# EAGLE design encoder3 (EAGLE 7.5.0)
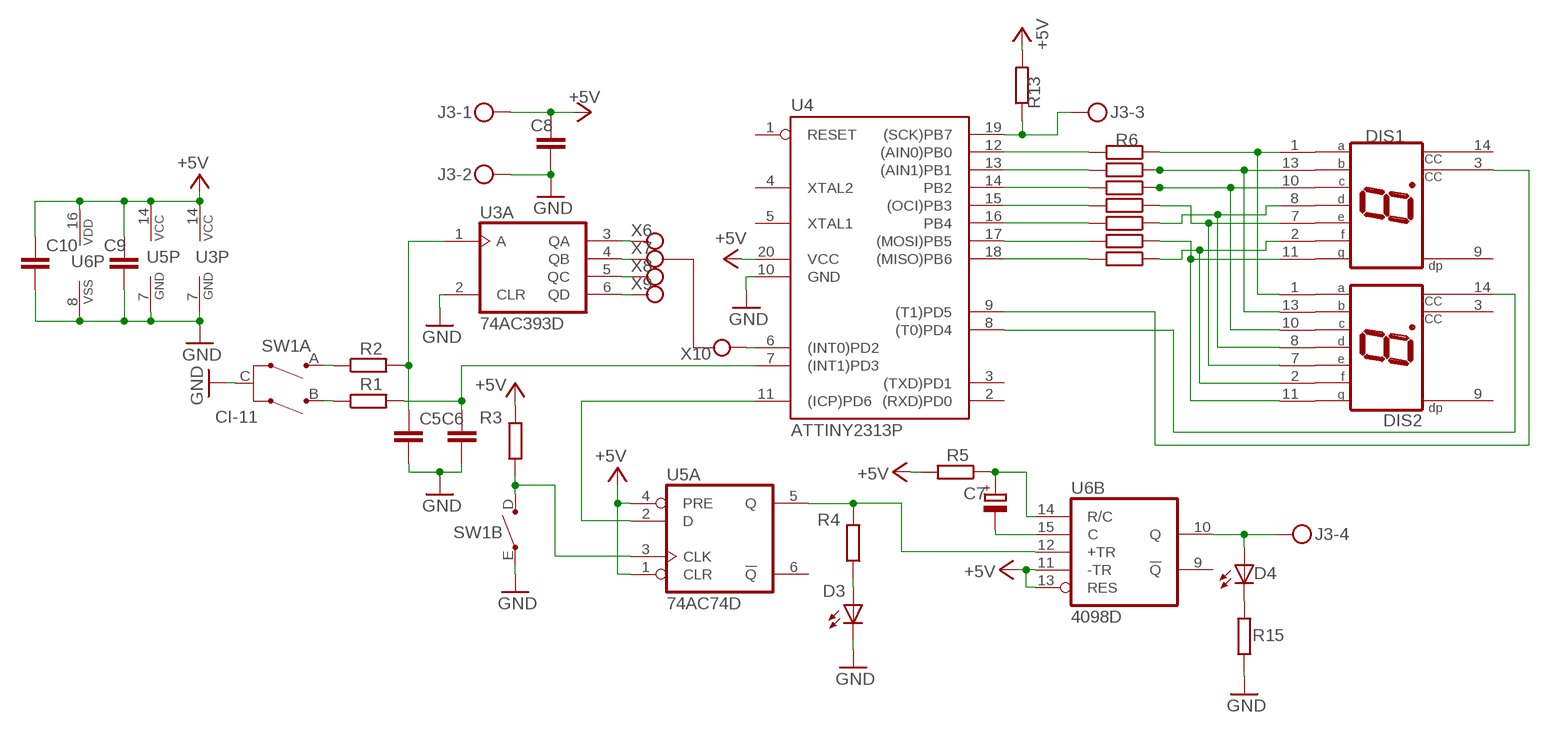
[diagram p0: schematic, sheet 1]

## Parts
C5  C-EUC1206  [C1206]
C6  C-EUC1206  [C1206]
C7  CPOL-EUE2.5-5  [E2,5-5]
C8  C-EUC1206  [C1206]
C9  C-EUC1206  [C1206]
C10  C-EUC1206  [C1206]
D3  LED3MM  [LED3MM]
D4  LED3MM  [LED3MM]
DIS1  VAOS-C402S9-BW/50  HD7740  [HD7730]
DIS2  VAOS-C402S9-BW/50  HD7740  [HD7730]
J3  MKDSN1,5/4-5,08  [MKDSN1,5/4-5,08]
R1  R-EU_0204/7  [0204/7]
R2  R-EU_0204/7  [0204/7]
R3  R-EU_0204/7  [0204/7]
R4  R-EU_0204/7  [0204/7]
R5  R-EU_0204/5  [0204/5]
R6  R-EU_0204/7  [0204/7]
R7  R-EU_0204/7  [0204/7]
R8  R-EU_0204/7  [0204/7]
R9  R-EU_0204/7  [0204/7]
R10  R-EU_0204/7  [0204/7]
R11  R-EU_0204/7  [0204/7]
R12  R-EU_0204/7  [0204/7]
R13  R-EU_0204/7  [0204/7]
R15  R-EU_0204/7  [0204/7]
SW1  CI-11  [CI-11]
U3  74AC393D  [SO14]
U4  ATTINY2313P  AT90S2313P  [DIL20]
U5  74AC74D  [SO14]
U6  4098D  [SO16]
X6  CONNWIRE  [CONNWIRE]
X7  CONNWIRE  [CONNWIRE]
X8  CONNWIRE  [CONNWIRE]
X9  CONNWIRE  [CONNWIRE]
X10  CONNWIRE  [CONNWIRE]

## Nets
+5V: C8.1 C9.1 C10.1 J3.1 R3.2 R5.2 R13.2 U3.14(P:VCC) U4.20(VCC) U5.1(A:CLR) U5.4(A:PRE) U5.14(P:VCC) U6.11(B:-TR) U6.13(B:RES) U6.16(P:VDD)
GND: C5.2 C6.2 C8.2 C9.2 C10.2 D3.K(C) J3.2 R15.1 SW1.C(A:C) SW1.E(B:E) U3.2(A:CLR) U3.7(P:GND) U4.10(GND) U5.7(P:GND) U6.8(P:VSS)
N$2: J3.3 R13.1 U4.19((SCK)PB7)
N$3: R2.1 SW1.A(A:A)
N$4: D4.A J3.4 U6.10(B:Q)
N$5: R1.1 SW1.B(A:B)
N$6: R6.2 U4.12((AIN0)PB0)
N$7: D4.K(C) R15.2
N$8: R7.2 U4.13((AIN1)PB1)
N$9: R8.2 U4.14(PB2)
N$10: R9.2 U4.15((OCI)PB3)
N$11: R10.2 U4.16(PB4)
N$12: DIS1.1(A) DIS2.1(A) R6.1
N$13: C6.1 R1.2 U4.7((INT1)PD3)
N$14: C5.1 R2.2 U3.1(A:A)
N$15: U3.3(A:QA) X6.P$1
N$16: U3.4(A:QB) X7.P$1
N$17: U3.5(A:QC) X8.P$1
N$18: U3.6(A:QD) X9.P$1
N$19: U4.6((INT0)PD2) X10.P$1
N$20: U4.11((ICP)PD6) U5.2(A:D)
N$21: R3.1 SW1.D(B:D) U5.3(A:CLK)
N$22: R12.2 U4.18((MISO)PB6)
N$23: DIS1.13(B) DIS2.13(B) R7.1
N$24: R4.2 U5.5(A:Q) U6.12(B:+TR)
N$25: D3.A R4.1
N$26: C7.+ R5.1 U6.14(B:R/C)
N$27: C7.- U6.15(B:C)
N$28: DIS1.10(C) DIS2.10(C) R8.1
N$29: DIS1.7(E) DIS2.7(E) R9.1
N$30: DIS1.8(D) DIS2.8(D) R10.1
N$32: DIS1.11(G) DIS2.11(G) R11.1
N$33: DIS1.2(F) DIS2.2(F) R12.1
N$34: R11.2 U4.17((MOSI)PB5)
N$35: DIS2.14(CC) U4.8((T0)PD4)
N$51: DIS1.3(CC) U4.9((T1)PD5)
Unconnected: DIS1.9(DP) DIS1.14(CC) DIS2.3(CC) DIS2.9(DP) U3.8(B:QD) U3.9(B:QC) U3.10(B:QB) U3.11(B:QA) U3.12(B:CLR) U3.13(B:A) U4.1(RESET) U4.2((RXD)PD0) U4.3((TXD)PD1) U4.4(XTAL2) U4.5(XTAL1) U5.6(A:!Q) U5.8(B:!Q) U5.9(B:Q) U5.10(B:PRE) U5.11(B:CLK) U5.12(B:D) U5.13(B:CLR) U6.1(A:C) U6.2(A:R/C) U6.3(A:RES) U6.4(A:+TR) U6.5(A:-TR) U6.6(A:Q) U6.7(A:!Q) U6.9(B:!Q)

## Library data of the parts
C5 C6 C8-C10 = rcl:C-EU: CAPACITOR, European symbol
C7 = rcl:CPOL-EU: POLARIZED CAPACITOR, European symbol
D3 D4 = led:LED: LED
DIS1 DIS2 = display-hp:HD7740: LED DISPLAY 1-character 7 segment, decimal point right; OC_FARNELL: unknown; OC_NEWARK: unknown
J3 = con-phoenix-508:MKDSN1,5/4-5,08: MKDSN 1,5/ 4-5,08 Printklemme Nennstrom: 13,5 A Nennspannung: 250 V Rastermaß: 5,08 mm Polzahl: 4 Anschlussart: Schraubanschluss Montage: Löten Anschlussrichtung Leiter/Platine: 0 ° Artikelnummer: 1729144 Source: http://eshop.phoenixcontact.com .. 1729144.pdf
R1-R13 R15 = rcl:R-EU_: RESISTOR, European symbol
SW1 = piher:CI-11: 11mm Incemental Encoder Source: www.piher.net .. 04-CI-11v04.pdf; OC_FARNELL: unknown; OC_NEWARK: unknown
U3 = 74xx-eu:74*393: Dual 4-bit decade and binary COUNTER
U4 = atmel:AT90S2313: MICROCONTROLLER 2 Kbytes FLASH 128 bytes SRAM 128 bytes EEPROM UART; OC_FARNELL: unknown; OC_NEWARK: unknown
U5 = 74xx-eu:74*74: Dual D type positive edge triggered FLIP FLOP, preset and clear
U6 = 40xx:4098: Dual monostable MULTIVIBRATOR Source: Texas Instruments (Data sheet acquired frm Harris Semiconductor SCHS065) http://pdf1.alldatasheet.com/datasheet-pdf/view/26897/TI/CD4098.html
X6-X10 = connholes:CONNWIRE

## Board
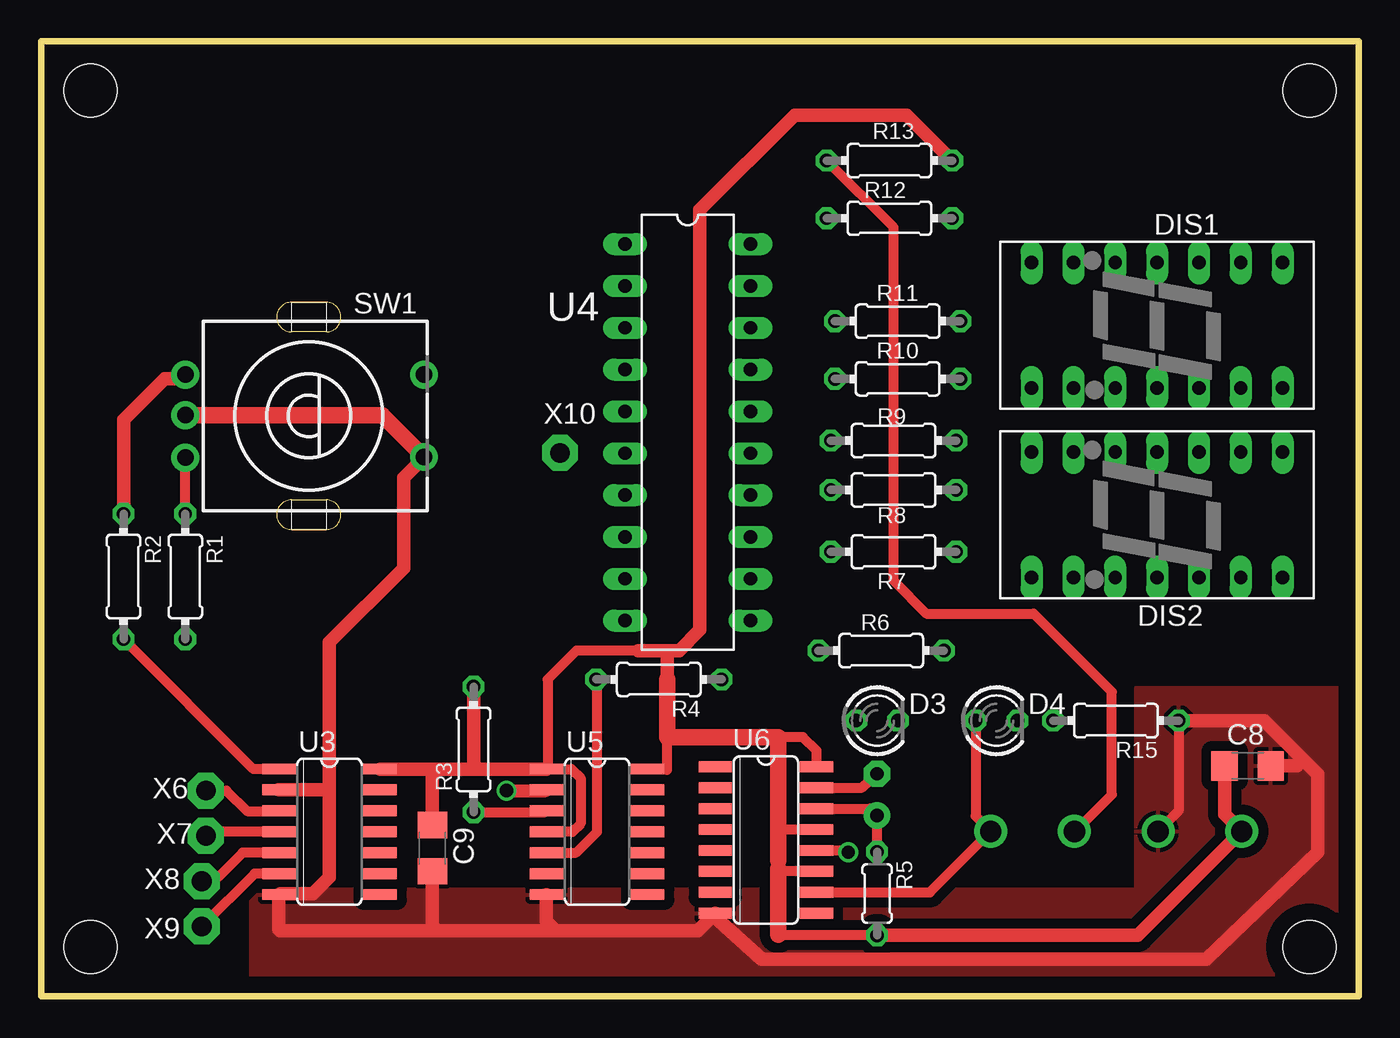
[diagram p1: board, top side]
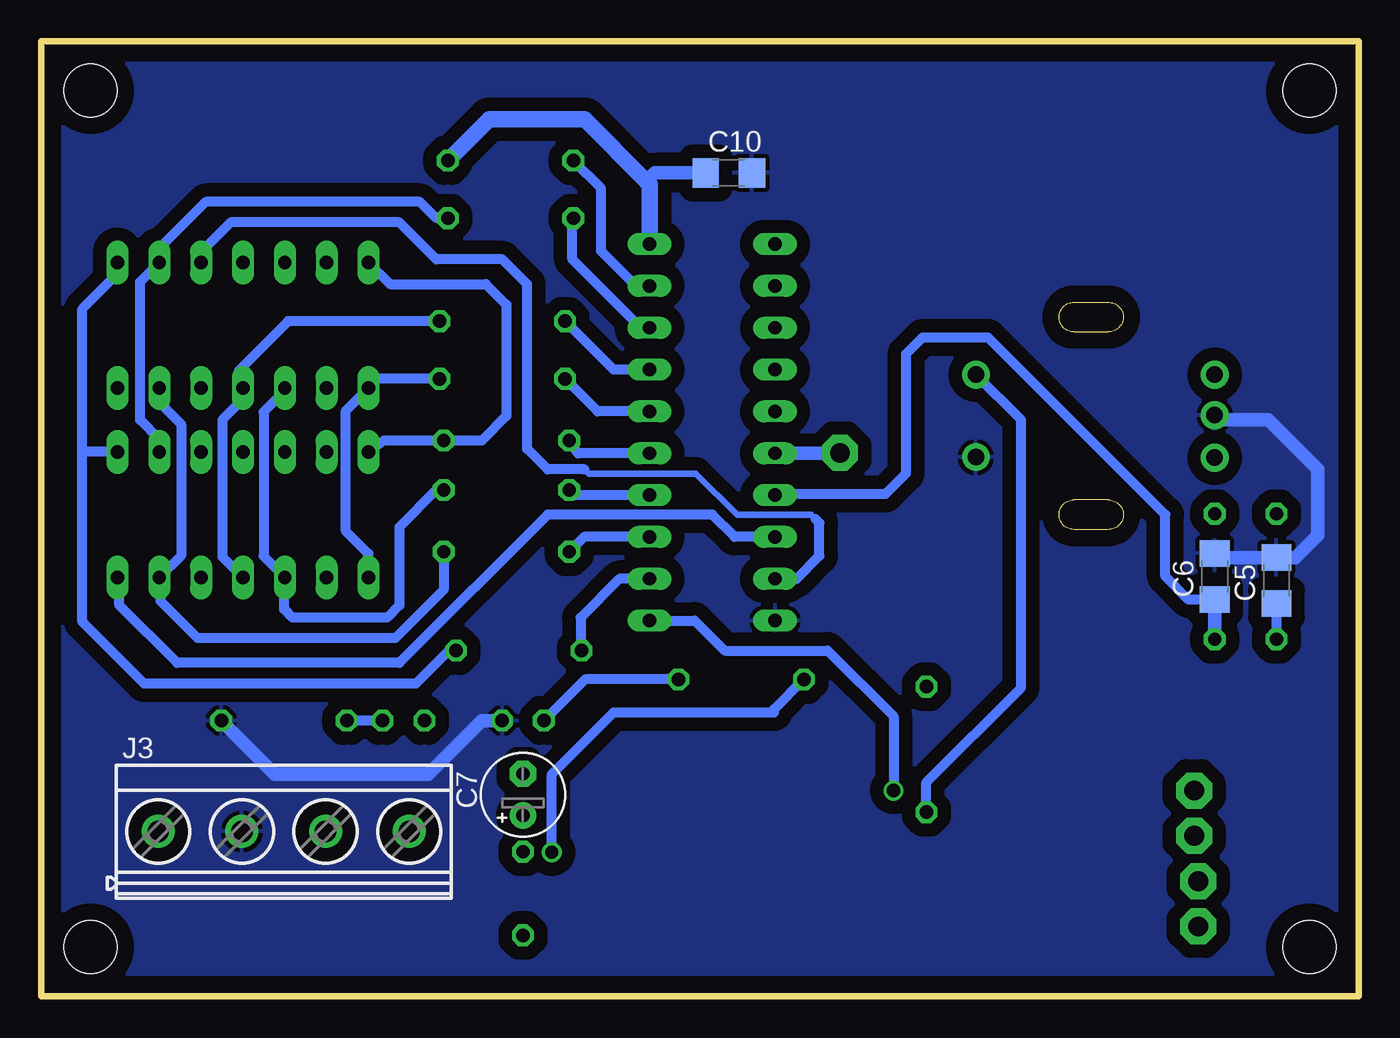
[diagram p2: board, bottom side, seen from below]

Size 80 x 58 mm. Coordinates in mm from the lower left corner, seen from the top.
Outline: 0,0 0,58 80,58 80,0 0,0
Copper layers (1*16): Top 0.035mm / dielectric 1.5mm / Bottom 0.035mm
Design rules "default": minimum track width 10mil, minimum drill 24mil, track to track 8mil, track to pad 8mil, pad to pad 8mil, via to via 8mil, smd to smd 8mil, copper to edge 40mil, drill to drill 8mil, minimum pad ring 10mil, minimum via ring 8mil, stop-mask expansion 4mil, vias tented up to drill 0mil, thermal gap 10mil
Holes 3.2 mm at 3,3 3,55 77,55 77,3

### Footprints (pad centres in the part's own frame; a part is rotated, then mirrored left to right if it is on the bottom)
C1206 = smd 1.6 x 1.8: 1 -1.4,0; 2 1.4,0
E2,5-5 = drill 0.813 pad 1.6: + -1.27,0 | drill 0.813 pad 1.6 octagon: - 1.27,0
LED3MM = drill 0.813 octagon: A -1.27,0; K 1.27,0
HD7730 = drill 0.813 long: 1 -3.81,7.62; 2 -3.81,5.08; 3 -3.81,2.54; 4 -3.81,0; 5 -3.81,-2.54; 6 -3.81,-5.08; 7 -3.81,-7.62; 8 3.81,-7.62; 9 3.81,-5.08; 10 3.81,-2.54; 11 3.81,0; 12 3.81,2.54; 13 3.81,5.08; 14 3.81,7.62
MKDSN1,5/4-5,08 = drill 1.3 pad 2: 1 -7.641,0.025; 2 -2.561,0.025; 3 2.519,0.025; 4 7.599,0.025
0204/7 = drill 0.813 octagon: 1 -3.81,0; 2 3.81,0
0204/5 = drill 0.813 octagon: 1 -2.54,0; 2 2.54,0
CI-11 = drill 1 pad 1.676: A -2.5,-7.5; B 2.54,-7.5; C -0.04,-7.5; D -2.5,7; E 2.5,7
SO14 = smd 0.66 x 2.032: 1 -3.81,-3.073; 2 -2.54,-3.073; 3 -1.27,-3.073; 4 0,-3.073; 5 1.27,-3.073; 6 2.54,-3.073; 7 3.81,-3.073; 8 3.81,3.073; 9 2.54,3.073; 10 1.27,3.073; 11 0,3.073; 12 -1.27,3.073; 13 -2.54,3.073; 14 -3.81,3.073
DIL20 = drill 0.813 long: 1 -11.43,-3.81; 2 -8.89,-3.81; 3 -6.35,-3.81; 4 -3.81,-3.81; 5 -1.27,-3.81; 6 1.27,-3.81; 7 3.81,-3.81; 8 6.35,-3.81; 9 8.89,-3.81; 10 11.43,-3.81; 11 11.43,3.81; 12 8.89,3.81; 13 6.35,3.81; 14 3.81,3.81; 15 1.27,3.81; 16 -1.27,3.81; 17 -3.81,3.81; 18 -6.35,3.81; 19 -8.89,3.81; 20 -11.43,3.81
SO16 = smd 0.66 x 2.032: 1 -4.445,-3.073; 2 -3.175,-3.073; 3 -1.905,-3.073; 4 -0.635,-3.073; 5 0.635,-3.073; 6 1.905,-3.073; 7 3.175,-3.073; 8 4.445,-3.073; 9 4.445,3.073; 10 3.175,3.073; 11 1.905,3.073; 12 0.635,3.073; 13 -0.635,3.073; 14 -1.905,3.073; 15 -3.175,3.073; 16 -4.445,3.073
CONNWIRE = drill 1.2 pad 2.184 octagon: P$1 0,0

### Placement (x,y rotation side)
C5  5,25.25 90 bottom
C6  8.75,25.5 90 bottom
C7  50.75,12.25 90 bottom
C8  73.25,14 0 top
C9  23.75,9 270 top
C10  38.25,50 0 bottom
D3  50.75,16.75 0 top
D4  58,16.75 0 top
DIS1  67.75,40.75 270 top
DIS2  67.75,29.25 270 top
J3  65.25,10 0 bottom
R1  8.75,25.5 270 top
R2  5,25.5 270 top
R3  26.25,15 90 top
R4  37.5,19.25 180 top
R5  50.75,6.25 270 top
R6  51,21 180 top
R7  51.75,27 180 top
R8  51.75,30.75 180 top
R9  51.75,33.75 180 top
R10  52,37.5 180 top
R11  52,41 180 top
R12  51.5,47.25 180 top
R13  51.5,50.75 0 top
R15  65.25,16.75 180 top
SW1  16.25,35.25 270 top
U3  17.5,10 270 top
U4  39.25,34.25 270 top
U5  33.75,10 270 top
U6  44,9.5 270 top
X6  10,12.5 0 top
X7  10,9.75 0 top
X8  9.75,7 0 top
X9  9.75,4.25 0 top
X10  31.5,33 0 top

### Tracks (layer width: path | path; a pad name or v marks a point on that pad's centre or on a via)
+5V
  Top 0.61: U6.16 47.07,14.93 46.25,15.75 44.75,15.75 | 38,15.75 38.25,15.75 38,15.5 38,13.75 37.94,13.81 U5.14 | 36.25,21 32.5,21 30.75,19.25 30.75,13.88 U5.1 32.19,13.81 32.75,13.25 32.75,10.5 32.25,10 U5.4 | U6.11 44.91,7.59 44.75,7.75 44.75,8 44.88,8.12 44.75,8.25 | U6.13 44.88,10.13 44.75,10 | R5.2 44.79,3.71 44.75,3.75
  Top 0.813: 36.25,21 38.25,21 | 38.25,21 38.75,21 40,22.25 40,47.75 45.75,53.5 52.56,53.5 R13.2 | 38,19.25 38,20.75 38.25,21 | U3.14 24,13.81 | 24,13.81 26.5,13.81 | 26.5,13.81 U5.1 | R3.2 26.25,14.06 26.5,13.81 | R5.2 66.58,3.71 J3.1 71.85,11.07 C8.1 | C9.1 23.75,13.56 24,13.81
  Top 1: 44.75,15.75 38.25,15.75
  Top 1.016: 38,15.75 38,19.25 | 44.75,8.25 44.75,10 44.75,15.75 | 44.75,3.75 44.75,7.75
  Bottom 0.61: 43.06,49.31 43.25,49.5
  Bottom 0.813: C10.1 42.75,50 43.25,49.5
  Bottom 1.016: U4.20 43.06,49.31 | 43.25,49.5 47,53.25 52.81,53.25 R13.2
GND
  Top 0.61: R15.1 69.06,11.27 J3.2 | U3.7 14.5,6.25
  Top 0.813: U3.7 14.43,4.07 14.5,4 24,4 | 24,4 31.25,4 | 31.25,4 39.87,4 U6.8 40.93,4.82 43.75,2.25 70.75,2.25 77.5,8.75 77.5,13.5 76.62,14.38 | U5.7 30.68,4.57 31.25,4 | 14.5,6.25 16.5,6.25 17.5,7.25 17.5,12.5 | U3.2 17.46,12.54 17.5,12.5 | 76.62,14.38 74.25,16.75 R15.1 | C9.2 23.75,4.25 24,4 | C8.2 76.25,14 76.62,14.38 | 17.5,12.5 17.5,21.5 22,26 22,31.5 SW1.E
  Top 1.016: SW1.C 20.71,35.29 SW1.E
  Bottom 0.813: D3.K 53.25,16.75 56.5,13.5 65.81,13.5 R15.1 | SW1.C 8.46,35 5.5,35 2.5,32 2.5,28 3.85,26.65 C5.2 8.5,26.65 C6.2
  pour Bottom (isolate 0.813): 0.25,57.5 79.5,57.5 79.5,0.75 0.25,0.75
  pour Top (isolate 0.61): 12.75,6.5 66.5,6.5 66.5,18.75 79.75,18.75 79.75,0.5 12.75,0.5
N$2
  Top 0.61: J3.3 62.77,10.03 65,12.25 65,18.5 60.25,23.25 53.75,23.25 51.75,25.25 51.75,46.69 R13.1
  Bottom 0.61: U4.19 43.89,43.14 46,45.25 46,49.06 R13.1
N$3
  Top 0.813: R2.1 5,35 7.5,37.5 8.5,37.5 SW1.A
N$4
  Top 0.61: 57.5,9.87 J3.4 | D4.A 56.73,10.95 J3.4 | U6.10 53.95,6.33 J3.4
N$5
  Top 0.61: R1.1 SW1.B
N$6
  Bottom 0.61: U4.12 44.89,25.36 47.25,23 47.25,21.06 R6.2
N$7
  Bottom 0.61: D4.K R15.2
N$8
  Bottom 0.61: U4.13 47.04,27.9 R7.2
N$9
  Bottom 0.61: U4.14 47.63,30.44 R8.2
N$10
  Bottom 0.61: U4.15 47.42,32.98 R9.2
N$11
  Bottom 0.61: U4.16 46.21,35.52 R10.2
N$12
  Bottom 0.61: DIS1.1 75.37,43.88 77.5,41.75 77.5,33.25 | 77.5,33.25 77.5,22.75 73.75,19 57.25,19 55.25,21 R6.1 | DIS2.1 77.31,33.06 77.5,33.25
N$13
  Bottom 0.61: C6.1 10.35,24.1 11.75,25.5 11.75,29.25 22.5,40 26.5,40 27.5,39 27.5,31.75 28.75,30.5 35.38,30.5 U4.7
  Bottom 0.813: C6.1 R1.2
N$14
  Top 0.61: U3.1 12.88,13.81 R2.2
  Bottom 0.61: C5.1 R2.2
N$15
  Top 0.61: X6.P$1 11.25,12.5 12.5,11.25 14.41,11.25 U3.3
N$16
  Top 0.61: U3.4 10.25,10 X7.P$1
N$17
  Top 0.61: U3.5 12.23,8.73 10.75,7.25 10,7.25 X8.P$1
N$18
  Top 0.61: U3.6 12.96,7.46 X9.P$1
N$19
  Bottom 0.813: U4.6 31.52,32.98 X10.P$1
N$20  (via drill 0.8)
  Top 0.61: 30.64,12.5 U5.2
  Top 0.8: v28.25,12.5 30.64,12.5
  Bottom 0.61: U4.11 40.32,22.82 38.5,21 32.25,21 28.25,17 v28.25,12.5
N$21
  Top 0.61: R3.1 30.6,11.19 U5.3
  Bottom 0.61: R3.1 26.25,13 20.5,18.75 20.5,35 SW1.D
N$22
  Bottom 0.61: U4.18 43.6,40.6 47.75,44.75 47.75,47.19 R12.2
N$23
  Bottom 0.61: DIS1.13 72.83,36.08 71.5,34.75 71.5,26.77 DIS2.13 72.75,25.36 72.75,24 70.5,21.75 58.5,21.75 55.56,24.69 R7.1
N$24  (via drill 0.8)
  Top 0.61: U6.12 48.88,8.87 v49,8.75 | U5.5 32.48,8.73 33.75,10 33.75,19.19 R4.2
  Bottom 0.61: v49,8.75 49,13.5 45.25,17.25 35.5,17.25 35.5,17.44 R4.2
N$25
  Bottom 0.61: R4.1 46.98,19.25 D3.A
N$26
  Top 0.61: U6.14 50.33,11.4 C7.+ R5.1
N$27
  Top 0.61: U6.15 49.84,12.68 C7.-
N$28
  Bottom 0.61: DIS1.10 65.21,36.79 66.5,35.5 66.5,26.73 DIS2.10 65.25,25.4 65.25,23.5 64.75,23 59,23 58.25,23.75 58.25,28.5 56,30.75 R8.1
N$29
  Bottom 0.61: DIS2.7 59.19,33.75 R9.1 53.25,33.75 51.75,35.25 51.75,42 53,43.25 58.82,43.25 DIS1.7
N$30
  Bottom 0.61: DIS2.8 60.13,26.88 61.5,28.25 61.5,35.57 DIS1.8 59.57,37.5 R10.1
N$32
  Bottom 0.61: R11.1 65,41 68,38 68,37.19 DIS1.11 67.75,36.25 69,35 69,26.69 DIS2.11
N$33
  Bottom 0.61: R12.1 56,47.25 57,48.25 70,48.25 73,45.25 73,44.73 DIS1.2 74,43.39 74,35 72.83,33.83 DIS2.2
N$34
  Bottom 0.61: U4.17 45.25,38.06 R11.2
N$35
  Bottom 0.61: U4.8 37.9,27.9 39.25,29.25 49.25,29.25 58.25,20.25 71.75,20.25 75.25,23.75 75.25,25.32 DIS2.14
N$51
  Bottom 0.406: 33,29 33.25,29.25 37.75,29.25 40.25,31.75 46.75,31.75 47,32
  Bottom 0.61: U4.9 34.14,25.36 32.75,26.75 32.75,28.75 33,29 | 47,32 49.25,32 50.5,33.25 50.5,43.25 52,44.75 56,44.75 58.25,47 68.5,47 70.25,45.25 70.25,44.6 DIS1.3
